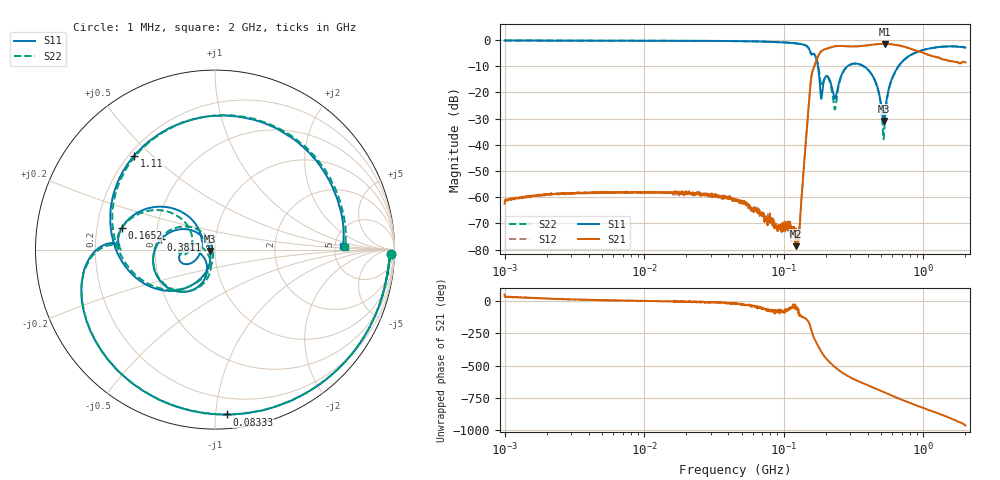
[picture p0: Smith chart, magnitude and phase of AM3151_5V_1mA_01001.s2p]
! Date/Time: Fri Jun 26 10:43:32 2020
! Network Analyzer:  Rev:
! Sweep from 1000000.0 to 2000000000.0, 1601 Points ! Power Supply: 0 V, 0 A
# HZ S DB R 50
!freq MagS11 AngS11 MagS21 AngS21 MagS12 AngS12 MagS22 AngS22
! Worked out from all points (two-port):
!   1601 points, 1 MHz to 2 GHz, reference 50 ohm
!   highest |S21| = -1.46 dB at 531.4 MHz (marker M1); lowest = -78.7 dB at 123 MHz (marker M2)
!   |S21| within 3 dB of the highest: 184.2 MHz to 946.7 MHz (762.5 MHz wide, 135 % of centre)
!   lowest |S11| = -30.9 dB at 518.9 MHz (marker M3), VSWR 1.06, Z = 47.3 - j0.672 ohm
!   |S11| at or under -10 dB: 175.6 MHz to 285.6 MHz (110 MHz wide, 47.7 % of centre); 373.7 MHz to 662.7 MHz (288.9 MHz wide, 55.8 % of centre)
!   |S22| runs from -37.8 to -0.2 dB; largest |S21 - S12| = 0.009
!   S11 on the Smith chart (normalised r, x): 1 MHz: 35, -48; 83.33 MHz: 0.09, -1.07; 165.2 MHz: 0.31, +0.10; 381.1 MHz: 0.53, +0.07; 1.11 GHz: 0.22, +0.44; 2 GHz: 5.97, +0.52
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1000000  -0.17 -1.6  -62.43 51.3  -60.83 34.7  -0.17 -1.6
3555161  -0.24 -4.0  -58.27 11.4  -58.25 11.3  -0.24 -4.1
1.263916e7  -0.28 -13.4  -58.19 0.9  -58.15 0.4  -0.28 -13.3
4.493426e7  -0.41 -46.7  -61.03 -23.5  -61.35 -16.7  -0.42 -46.6
8.33271e7  -0.72 -85.9  -70.89 -67.2  -69.75 -82.4  -0.73 -85.9
1.230167e8  -1.28 -130.0  -78.66 -49.0  -75.45 -47.9  -1.29 -130.0
1.308532e8  -1.50 -140.4  -69.47 -105.8  -68.78 -120.6  -1.48 -140.2
1.589914e8  -5.47 177.7  -12.83 120.6  -12.81 120.5  -5.55 -179.8
1.651501e8  -5.46 166.9  -10.09 71.3  -10.09 71.3  -5.30 170.5
1.833445e8  -20.19 139.7  -4.59 -22.1  -4.58 -22.0  -16.05 146.3
2.074482e8  -14.00 -171.1  -3.14 -101.1  -3.14 -101.1  -14.38 175.1
2.325012e8  -22.38 -145.7  -2.41 -152.0  -2.40 -152.0  -26.55 -146.5
2.556749e8  -14.17 -110.9  -2.27 173.2  -2.28 173.0  -14.48 -107.3
3.810586e8  -10.28 169.3  -2.14 76.3  -2.13 76.6  -10.32 166.0
4.586222e8  -16.50 138.0  -1.62 39.6  -1.61 39.6  -16.62 130.8
5.189154e8  -30.89 -165.6  -1.47 14.6  -1.48 14.5  -37.85 -167.8
5.313877e8  -27.30 -125.3  -1.46 9.7  -1.47 9.7  -29.43 -108.3
5.652395e8  -18.65 -110.9  -1.56 -2.9  -1.54 -3.0  -18.97 -105.7
7.69728e8  -6.46 -162.0  -2.92 -63.2  -2.93 -63.2  -6.53 -164.0
1.109683e9  -3.23 130.6  -5.81 -127.2  -5.79 -127.3  -3.20 127.2
1.482693e9  -2.44 73.1  -7.77 -179.2  -7.66 -179.6  -2.38 70.2
2e9  -2.91 1.7  -8.52 115.1  -8.67 114.5  -2.78 1.3
